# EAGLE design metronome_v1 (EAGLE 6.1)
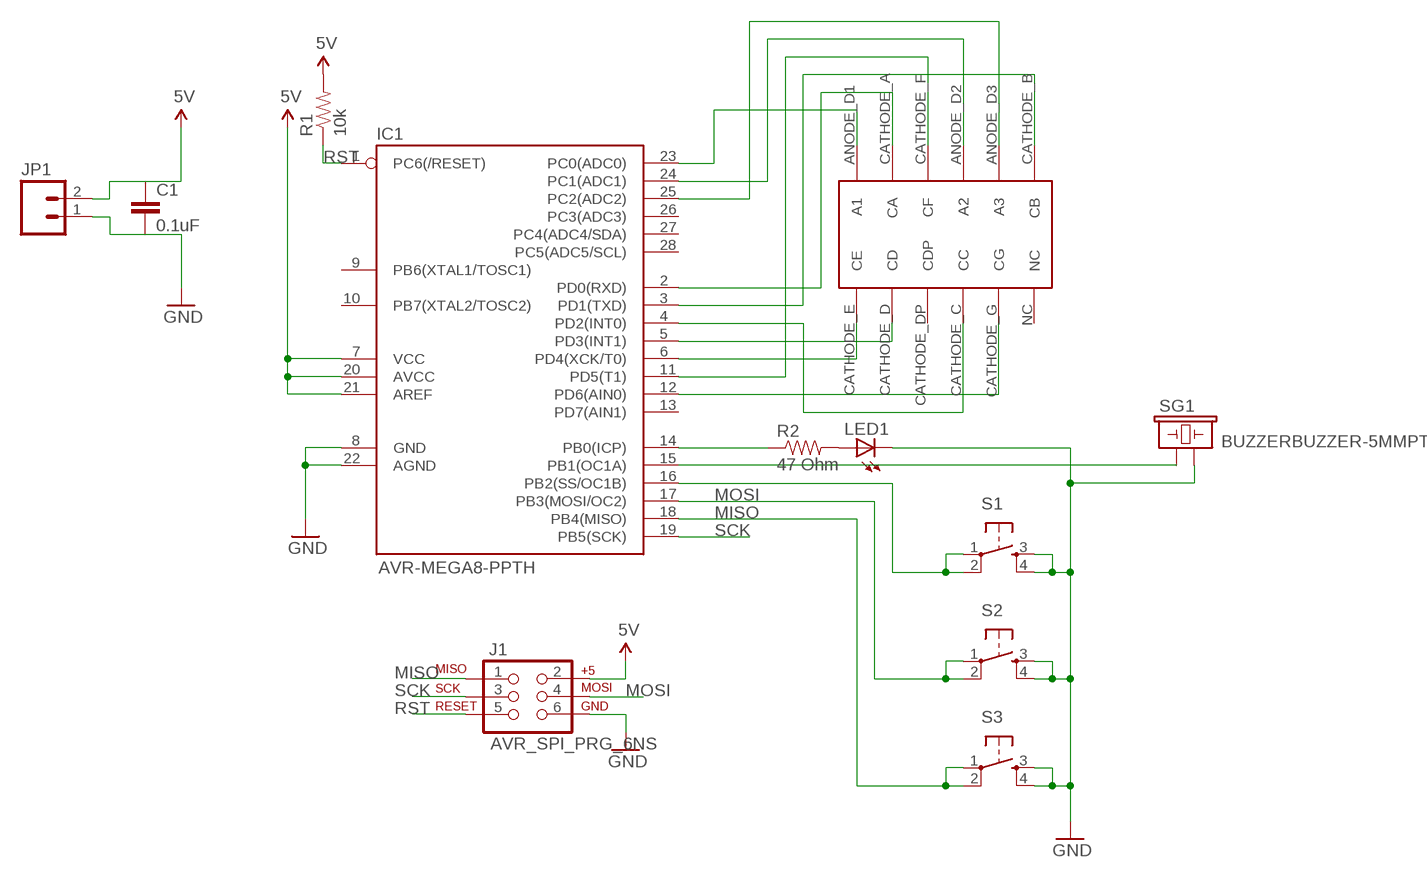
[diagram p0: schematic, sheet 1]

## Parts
C1  0.1uF  CAPPTH  [CAP-PTH-SMALL]
IC1  AVR-MEGA8-PPTH  [DIL28-3]
J1  AVR_SPI_PRG_6NS  [2X3-NS]
JP1  M02PTH3  [1X02_LONGPADS]
LED1  LED5MM  [LED5MM]
R1  10k  RESISTORAXIAL-0.3  [AXIAL-0.3]
R2  47 Ohm  RESISTORAXIAL-0.3  [AXIAL-0.3]
S1  TAC_SWITCHPTH  [TACTILE-PTH]
S2  TAC_SWITCHPTH  [TACTILE-PTH]
S3  TAC_SWITCHPTH  [TACTILE-PTH]
SG1  BUZZERBUZZER-5MMPTH  [BUZZER-5MMPTH]
U$1  7-SEGMENT-3DIGIT-LTC516R  [7-SEGMENT-3DIGIT-LTC561R]

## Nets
5V: C1.1 IC1.7(VCC) IC1.20(AVCC) IC1.21(AREF) J1.2 JP1.2 R1.P$2
GND: C1.2 IC1.8(GND) IC1.22(AGND) J1.6 JP1.1 LED1.K(C) S1.3 S1.4 S2.3 S2.4 S3.3 S3.4 SG1.P$2
MISO: IC1.18(PB4(MISO)) J1.1 S3.1 S3.2
MOSI: IC1.17(PB3(MOSI/OC2)) J1.4 S2.1 S2.2
N$1: LED1.A R2.P$2
N$2: IC1.14(PB0(ICP)) R2.P$1
N$3: IC1.2(PD0(RXD)) U$1.CATHODE_A(CA)
N$4: IC1.3(PD1(TXD)) U$1.CATHODE_B(CB)
N$5: IC1.15(PB1(OC1A)) SG1.P$1
N$6: IC1.16(PB2(SS/OC1B)) S1.1 S1.2
N$9: IC1.4(PD2(INT0)) U$1.CATHODE_C(CC)
N$10: IC1.5(PD3(INT1)) U$1.CATHODE_D(CD)
N$11: IC1.6(PD4(XCK/T0)) U$1.CATHODE_E(CE)
N$12: IC1.11(PD5(T1)) U$1.CATHODE_F(CF)
N$13: IC1.12(PD6(AIN0)) U$1.CATHODE_G(CG)
N$14: IC1.23(PC0(ADC0)) U$1.ANODE_D1(A1)
N$15: IC1.24(PC1(ADC1)) U$1.ANODE_D2(A2)
N$16: IC1.25(PC2(ADC2)) U$1.ANODE_D3(A3)
RST: IC1.1(PC6(/RESET)) J1.5 R1.P$1
SCK: IC1.19(PB5(SCK)) J1.3
Unconnected: IC1.9(PB6(XTAL1/TOSC1)) IC1.10(PB7(XTAL2/TOSC2)) IC1.13(PD7(AIN1)) IC1.26(PC3(ADC3)) IC1.27(PC4(ADC4/SDA)) IC1.28(PC5(ADC5/SCL)) U$1.CATHODE_DP(CDP) U$1.NC

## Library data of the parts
C1 = SparkFun-Passives:CAP: Capacitor
IC1 = SparkFun-DigitalIC:AVR-MEGA8-P: MICROCONTROLLER 8 Kbytes FLASH 1 kbytes SRAM 512 bytes EEPROM USART 4-channel 10 bit ADC 2-channel 8 bit ADC
J1 = SparkFun-Connectors:AVR_SPI_PRG_6: AVR ISP 6 Pin This is the reduced ISP connector for AVR programming. Common on Arduino. This footprint will take up less PCB space and can be used with a 10-pin to 6-pin adapter such as SKU: BOB-08508
JP1 = SparkFun-Connectors:M02: Header 2
LED1 = SparkFun-LED:LED: LEDs
R1 R2 = SparkFun-Passives:RESISTOR: Resistor
S1-S3 = SparkFun-Electromechanical:TAC_SWITCH: Momentary Switch Button commonly used for reset or general input. Spark Fun Electronics SKU : COM-00097
SG1 = SparkFun-Electromechanical:BUZZER: Buzzer 12mm
U$1 = SparkFun-Displays:7-SEGMENT-3DIGIT-LTC516R

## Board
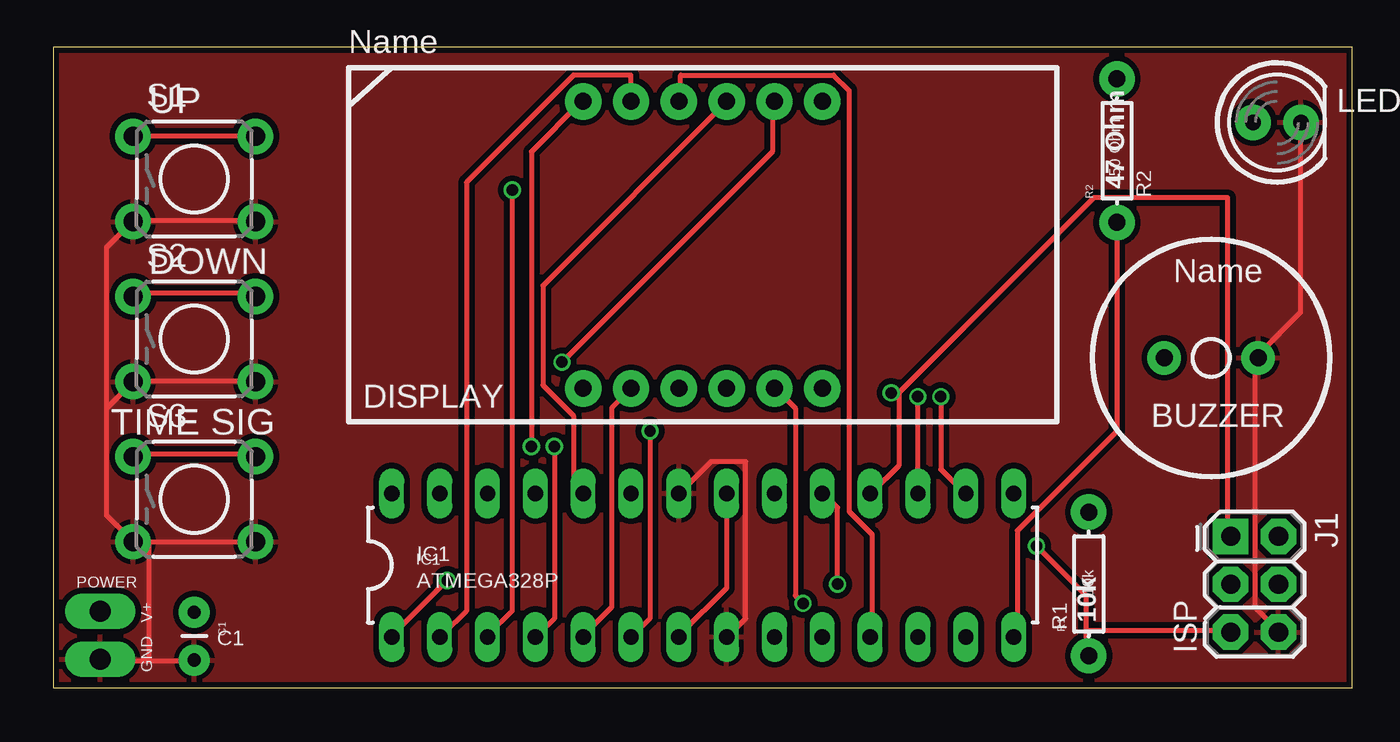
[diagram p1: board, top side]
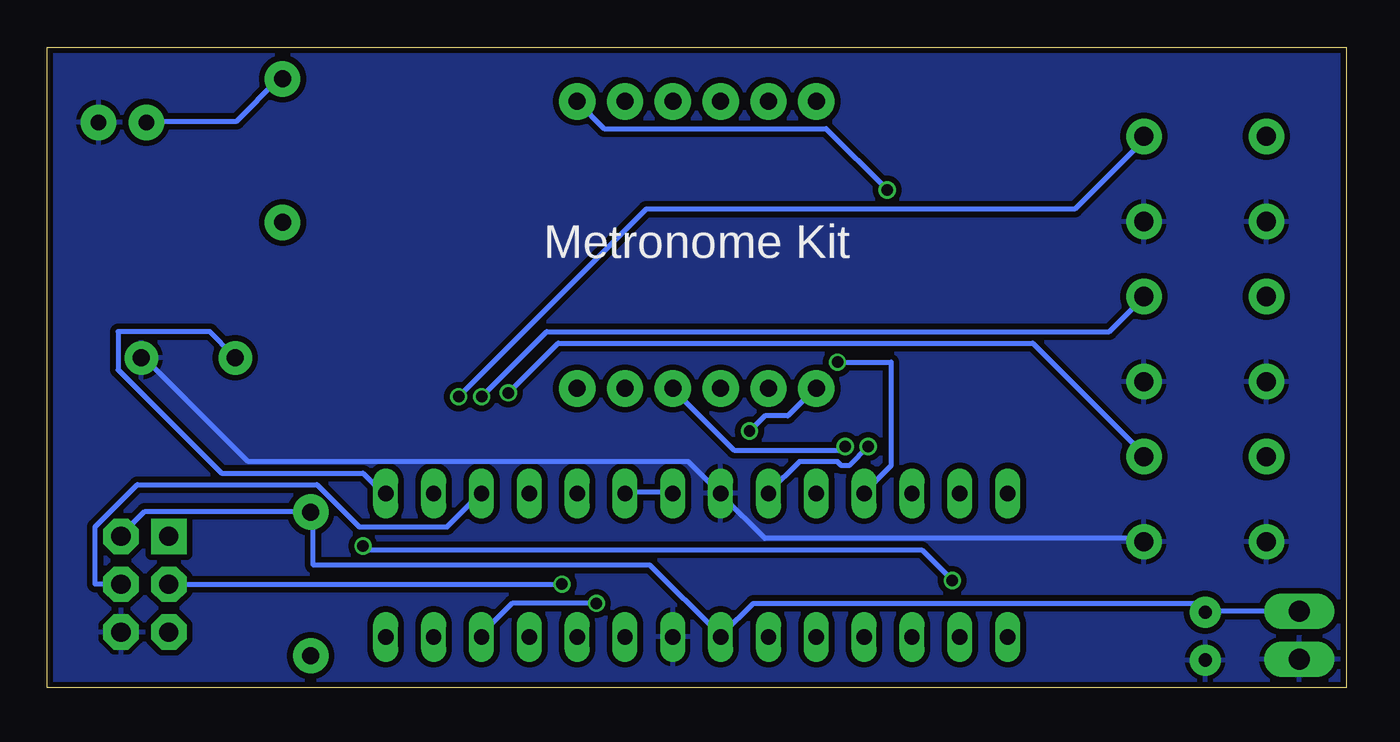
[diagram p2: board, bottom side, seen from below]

Size 69 x 34 mm. Coordinates in mm from the lower left corner, seen from the top.
Outline: 0,0 69,0 69,34 0,34 0,0
Copper layers (1*16): Top 0.035mm / dielectric 1.5mm / Bottom 0.035mm
Design rules: minimum track width 6mil, minimum drill 12mil, track to track 6mil, track to pad 6mil, pad to pad 6mil, via to via 6mil, smd to smd 0mil, copper to edge 10mil, drill to drill 10mil, minimum pad ring 10mil, minimum via ring 6mil, stop-mask expansion 2mil, vias tented up to drill 100mil, thermal gap 10mil

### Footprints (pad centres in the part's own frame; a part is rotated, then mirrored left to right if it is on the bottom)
CAP-PTH-SMALL = drill 0.7 pad 1.651: 1 0,0; 2 2.54,0
DIL28-3 = drill 0.813 long: 1 -16.51,-3.81; 2 -13.97,-3.81; 3 -11.43,-3.81; 4 -8.89,-3.81; 5 -6.35,-3.81; 6 -3.81,-3.81; 7 -1.27,-3.81; 8 1.27,-3.81; 9 3.81,-3.81; 10 6.35,-3.81; 11 8.89,-3.81; 12 11.43,-3.81; 13 13.97,-3.81; 14 16.51,-3.81; 15 16.51,3.81; 16 13.97,3.81; 17 11.43,3.81; 18 8.89,3.81; 19 6.35,3.81; 20 3.81,3.81; 21 1.27,3.81; 22 -1.27,3.81; 23 -3.81,3.81; 24 -6.35,3.81; 25 -8.89,3.81; 26 -11.43,3.81; 27 -13.97,3.81; 28 -16.51,3.81
2X3-NS = drill 1.016 pad 1.88 square: 1 -2.54,-1.27 | drill 1.016 pad 1.88 octagon: 2 -2.54,1.27; 3 0,-1.27; 4 0,1.27; 5 2.54,-1.27; 6 2.54,1.27
1X02_LONGPADS = drill 1.118 pad 1.88 long: 1 0,0; 2 2.54,0
LED5MM = drill 0.813 pad 1.88: A -1.27,0; K 1.27,0
AXIAL-0.3 = drill 0.9 pad 1.88: P$1 -3.81,0; P$2 3.81,0
TACTILE-PTH = drill 1.016 pad 1.88: 1 -3.251,2.261; 2 3.251,2.261; 3 -3.251,-2.261; 4 3.251,-2.261
BUZZER-5MMPTH = drill 0.9 pad 1.778: P$1 -2.5,0; P$2 2.5,0
7-SEGMENT-3DIGIT-LTC561R = drill 0.9 pad 1.93: ANODE_D1 -6.35,7.62; ANODE_D2 1.27,7.62; ANODE_D3 3.81,7.62; CATHODE_A -3.81,7.62; CATHODE_B 6.35,7.62; CATHODE_C 1.27,-7.62; CATHODE_D -3.81,-7.62; CATHODE_DP -1.27,-7.62; CATHODE_E -6.35,-7.62; CATHODE_F -1.27,7.62; CATHODE_G 3.81,-7.62; NC 6.35,-7.62

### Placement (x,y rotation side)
C1  7.5,4 270 top
IC1  34.5,6.5 0 top
J1  63.8,5.49 270 top
JP1  2.5,1.5 90 top
LED1  65,30 0 top
R1  55,5.5 90 top
R2  56.5,28.5 90 top
S1  7.5,27 0 top
S2  7.5,18.5 0 top
S3  7.5,10 0 top
SG1  61.5,17.5 0 top
U$1  34.5,23.5 0 top

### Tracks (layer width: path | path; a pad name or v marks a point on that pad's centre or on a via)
5V
  Top 0.254: IC1.7 33.33,2.85 35.76,5.28 35.76,10.16 IC1.21
  Bottom 0.254: J1.2 65.02,8.13 63.8,9.35 55.07,9.35 R1.P$2 54.86,9.14 54.86,6.5 36.98,6.5 33.33,2.85 IC1.7 33.12,2.85 31.5,4.47 7.92,4.47 7.52,4.06 C1.1 7.32,4.06 2.64,4.06 JP1.2 | IC1.20 38.2,10.36 35.97,10.36 IC1.21
GND
  Top 0.254: LED1.K 66.24,29.87 66.24,19.91 64.01,17.68 SG1.P$2 63.8,17.48 63.8,4.27 65.02,3.05 J1.6 | IC1.22 33.33,10.36 34.95,11.99 36.78,11.99 36.78,3.66 35.97,2.85 IC1.8 | S1.4 10.57,24.79 4.27,24.79 S1.3 4.06,24.59 2.85,23.37 2.85,14.83 | S2.4 10.57,16.26 4.27,16.26 S2.3 4.06,16.05 2.85,14.83 | 5.08,1.42 2.64,1.42 JP1.1 | 5.08,1.42 7.32,1.42 C1.2 | 5.08,7.72 10.57,7.72 S3.4 | 5.08,7.72 4.27,7.72 S3.3 | 5.08,7.72 5.08,1.42 | 5.08,7.72 S3.3 | 2.85,14.83 2.85,9.14 4.06,7.92 S3.3
  Bottom 0.254: S3.4 10.77,7.92 30.89,7.92 33.12,10.16 IC1.22 33.33,10.36 34.95,11.99 58.32,11.99 63.8,17.48 SG1.P$2
  pour Top (isolate 0.305): 0,34.01 69.01,34.01 69.01,0 0,0
  pour Bottom (isolate 0.305): 0,34.01 69.01,34.01 69.01,0 0,0
MISO  (via drill 0.61)
  Top 0.254: S3.1 4.27,12.39 10.57,12.39 S3.2 | 44.91,15.65 44.91,11.79 43.48,10.36 IC1.18 | 44.91,15.65 55.27,26.01 62.38,26.01 62.38,8.13 J1.1 | 44.91,15.65 v44.5,15.65
  Bottom 0.254: v44.5,15.65 41.86,18.29 16.66,18.29 10.77,12.39 S3.2
MOSI  (via drill 0.61)
  Top 0.254: S2.1 4.27,20.93 10.57,20.93 S2.2 | v45.92,15.44 45.92,10.36 IC1.17
  Bottom 0.254: J1.4 66.45,5.49 66.45,8.53 64.21,10.77 54.66,10.77 52.43,8.53 47.75,8.53 46.13,10.16 IC1.17 | v45.92,15.44 42.47,18.9 12.6,18.9 10.77,20.73 S2.2
N$1
  Bottom 0.254: R2.P$2 56.69,32.31 58.93,30.07 63.6,30.07 LED1.A
N$2
  Top 0.254: IC1.14 51.21,2.85 51.21,8.33 56.49,13.61 56.49,24.59 R2.P$1
N$3
  Top 0.254: IC1.2 20.73,2.85 21.95,4.06 21.95,26.82 27.64,32.51 30.68,32.51 30.68,31.29 U$1.CATHODE_A
N$4  (via drill 0.61)
  Top 0.254: v24.38,26.42 24.38,4.06 23.16,2.85 IC1.3
  Bottom 0.254: v24.38,26.42 27.64,29.67 39.42,29.67 40.84,31.09 U$1.CATHODE_B
N$5
  Bottom 0.254: IC1.15 51.21,10.36 52.22,11.38 59.74,11.38 65.23,16.87 65.23,18.9 60.35,18.9 59.13,17.68 SG1.P$1
N$6  (via drill 0.61)
  Top 0.254: v47.14,15.44 47.14,11.58 48.36,10.36 IC1.16 | S1.1 4.27,29.26 10.57,29.26 S1.2
  Bottom 0.254: v47.14,15.44 37.19,25.4 14.43,25.4 10.77,29.06 S1.2
N$9  (via drill 0.61)
  Top 0.254: v26.62,12.8 26.62,3.66 25.81,2.85 IC1.4
  Bottom 0.254: v26.62,12.8 26.82,12.6 32.51,12.6 35.76,15.85 U$1.CATHODE_C
N$10
  Top 0.254: IC1.5 28.25,2.85 29.67,4.27 29.67,14.83 30.68,15.85 U$1.CATHODE_D
N$11  (via drill 0.61)
  Top 0.254: v31.7,13.61 31.7,3.66 30.89,2.85 IC1.6
  Bottom 0.254: v31.7,13.61 30.89,14.43 29.67,14.43 28.25,15.85 U$1.CATHODE_E
N$12
  Top 0.254: IC1.11 43.48,2.85 43.48,8.13 42.27,9.35 42.27,31.7 41.45,32.51 33.33,32.51 33.33,31.29 U$1.CATHODE_F
N$13  (via drill 0.61)
  Top 0.254: v39.83,4.47 39.42,4.88 39.42,14.83 38.41,15.85 U$1.CATHODE_G
  Bottom 0.254: v39.83,4.47 44.3,4.47 45.92,2.85 IC1.12
N$14  (via drill 0.61)
  Top 0.254: v25.4,12.8 25.4,28.45 28.04,31.09 U$1.ANODE_D1
  Bottom 0.254: v25.4,12.8 26.42,11.79 26.82,11.79 27.03,11.99 29.06,11.99 30.68,10.36 IC1.23
N$15
  Top 0.254: IC1.24 28.04,10.36 27.64,10.77 27.64,14.43 26.01,16.05 26.01,21.34 35.76,31.09 U$1.ANODE_D2
N$16  (via drill 0.61)
  Top 0.254: v27.03,17.27 38.2,28.45 38.2,31.09 U$1.ANODE_D3
  Bottom 0.254: v27.03,17.27 24.18,17.27 24.18,11.79 25.6,10.36 IC1.25
RST  (via drill 0.61)
  Top 0.254: v20.93,5.69 18.09,2.85 IC1.1 | v52.22,7.52 54.86,4.88 54.86,3.05 | 54.86,3.05 54.86,1.83 R1.P$1 | 54.86,3.05 62.38,3.05 J1.5
  Bottom 0.254: v20.93,5.69 22.55,7.32 52.02,7.32 v52.22,7.52
SCK  (via drill 0.61)
  Top 0.254: v41.66,5.49 41.66,9.55 41.05,10.16 IC1.19
  Bottom 0.254: J1.3 v41.66,5.49

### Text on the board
_tsilk: UP | 150 Ohm | R2 | DOWN | DISPLAY | BUZZER | TIME SIG | IC1 | POWER | ATMEGA328P | 10k | V+ | C1 | R1 | ISP | GND
_bsilk: Metronome Kit

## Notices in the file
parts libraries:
SparkFun-Displays: Licensing: CC v3.0 Share-Alike You are welcome to use this library for commercial purposes.
